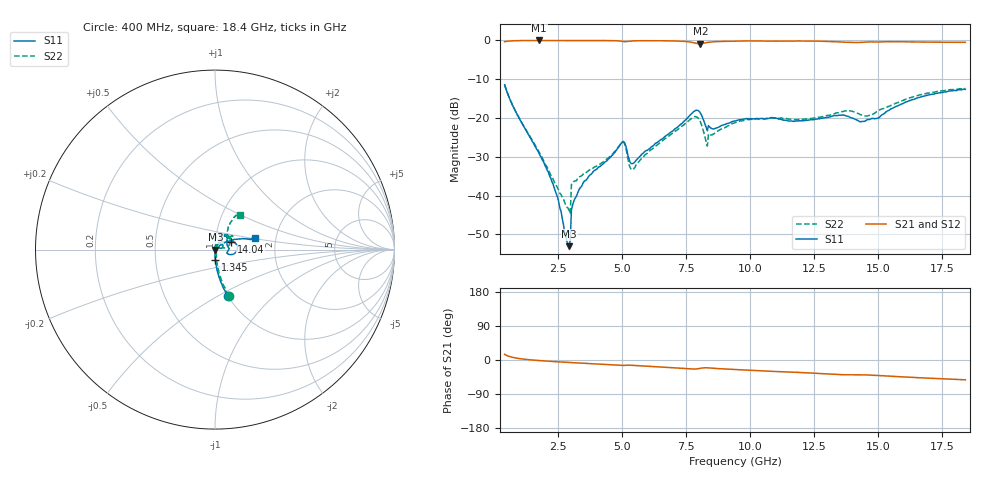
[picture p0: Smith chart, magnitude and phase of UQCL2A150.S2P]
! AVX Corporation
! Date:  10/27/06
! Part No:  UQCL2A150
! Description:  Ultra Low ESR Microwave capacitors
! Mounting Orientation:  Horizontal
# GHZ S DB R 50
! Freq  |S11|  S11 Ph  |S21|  S21 Ph  |S12|  S12 Ph  |S22|  S22 Ph
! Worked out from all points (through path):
!   401 points, 400 MHz to 18.4 GHz, reference 50 ohm
!   highest |S21| = -0.05 dB at 1.75 GHz (marker M1); lowest = -0.9 dB at 8.05 GHz (marker M2)
!   group delay of S21, straight-line fit = 8.42 ps
!   lowest |S11| = -53.0 dB at 2.92 GHz (marker M3), VSWR 1.00, Z = 50.2 - j0.0899 ohm
!   |S11| at or under -10 dB: start of sweep to end of sweep
!   |S22| runs from -44.7 to -11.4 dB; largest |S21 - S12| = 0.0075
!   S11 on the Smith chart (normalised r, x): 400 MHz: 1.00, -0.55; 1.345 GHz: 1.00, -0.12; 14.04 GHz: 1.19, +0.10; 18.4 GHz: 1.56, +0.21
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0.4  -11.49 -74.5  -0.37 14.8  -0.38 14.9  -11.43 -73.0
1.345  -24.42 -87.9  -0.07 0.8  -0.06 0.8  -24.29 -80.8
1.75  -29.20 -90.0  -0.05 -1.5  -0.05 -1.5  -28.80 -77.3
2.38  -38.86 -87.0  -0.06 -4.4  -0.05 -4.4  -37.21 -56.7
2.83  -51.74 -57.0  -0.06 -6.2  -0.06 -6.2  -42.92 -26.3
2.92  -53.03 -23.7  -0.06 -6.5  -0.06 -6.5  -43.77 -15.1
3.1  -41.50 113.3  -0.07 -7.2  -0.07 -7.2  -36.42 18.7
3.415  -37.53 96.8  -0.08 -8.3  -0.07 -8.3  -34.87 35.1
4.99  -26.21 41.4  -0.27 -14.4  -0.26 -14.3  -26.27 53.9
5.395  -31.79 28.5  -0.17 -14.1  -0.17 -14.0  -33.36 58.6
6.43  -25.96 38.7  -0.13 -18.2  -0.12 -18.1  -26.60 89.8
7.735  -18.71 20.0  -0.56 -24.0  -0.55 -23.9  -20.03 58.7
8.05  -18.75 -8.3  -0.91 -21.8  -0.88 -21.7  -21.05 22.0
8.23  -21.65 -18.8  -0.67 -20.5  -0.67 -20.5  -25.02 10.1
8.32  -23.32 -16.8  -0.55 -20.6  -0.54 -20.5  -27.25 13.1
9.4  -20.82 41.8  -0.23 -25.1  -0.22 -24.9  -21.22 69.8
12.415  -20.44 57.9  -0.21 -34.8  -0.21 -34.6  -20.10 37.9
14.035  -20.18 24.6  -0.58 -39.0  -0.57 -38.7  -18.42 34.7
14.62  -20.42 26.0  -0.43 -39.8  -0.42 -39.7  -19.38 47.0
15.43  -17.98 26.8  -0.38 -42.5  -0.37 -42.4  -16.98 59.0
16.78  -14.40 18.1  -0.46 -47.3  -0.45 -47.1  -13.85 59.5
18.4  -12.64 16.1  -0.52 -52.3  -0.52 -52.1  -12.44 54.3
